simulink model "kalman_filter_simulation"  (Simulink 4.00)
settings: Solver=VariableStepDiscrete  StartTime=0.0  StopTime=100.0  RelTol=1e-3
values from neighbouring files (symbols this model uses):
  A = [1.1269   -0.4940    0.1129    [Kalman_Filter_Design_Example.m]
  Akf = kalmf.a    [Kalman_Filter_Design_Example.m]
  Ao = A - Ko*C    [Kalman_Filter_Design_Example.m]
  B = [-0.3832    [Kalman_Filter_Design_Example.m]
  Bkf = kalmf.b    [Kalman_Filter_Design_Example.m]
  Bo = [B Ko]    [Kalman_Filter_Design_Example.m]
  C = [1 0 0]    [Kalman_Filter_Design_Example.m]
  Ckf = kalmf.c    [Kalman_Filter_Design_Example.m]
  Co = C    [Kalman_Filter_Design_Example.m]
  D = zeros(1,2)    [Kalman_Filter_Design_Example.m]
  Dkf = kalmf.d    [Kalman_Filter_Design_Example.m]
  Do = zeros(1,2)    [Kalman_Filter_Design_Example.m]
  Tc = 1    [Kalman_Filter_Design_Example.m]

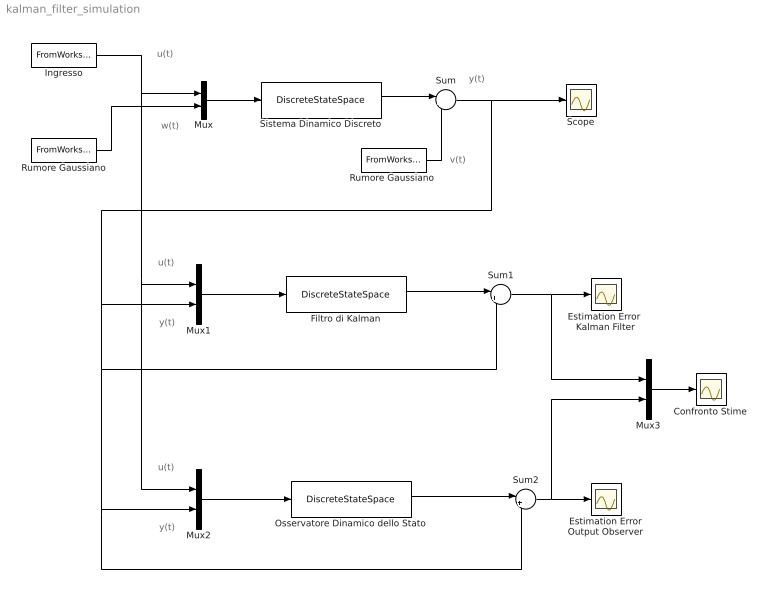
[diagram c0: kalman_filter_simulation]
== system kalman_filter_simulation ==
  note: u(t)
  note: w(t)
  note: y(t)
  note: v(t)
  note: u(t)
  note: y(t)
  note: u(t)
  note: y(t)
  Confronto Stime : Scope
  Estimation Error Output Observer : Scope
  Estimation Error  Kalman Filter : Scope
  Filtro di Kalman : DiscreteStateSpace  A=Akf  B=Bkf  C=Ckf  D=Dkf  X0=0  SampleTime=Tc  Realization=auto
  Ingresso : FromWorkspace  VariableName=[t u]  SampleTime=0  OutputAfterFinalValue=Extrapolation
  Mux{,1..3} (4 alike) : Mux  Inputs=2
  Osservatore Dinamico dello Stato : DiscreteStateSpace  A=Ao  B=Bo  C=Co  D=Do  X0=0  SampleTime=Tc  Realization=auto
  Rumore Gaussiano : FromWorkspace  VariableName=[t w]  SampleTime=Tc  OutputAfterFinalValue=Extrapolation
  "Rumore Gaussiano " : FromWorkspace  VariableName=[t v]  SampleTime=Tc  OutputAfterFinalValue=Extrapolation
  Scope : Scope
  Sistema Dinamico Discreto : DiscreteStateSpace  A=A  B=[B B]  C=C  D=D  X0=0  SampleTime=Tc  Realization=auto
  Sum : Sum  Inputs=|++  SaturateOnIntegerOverflow=on
  Sum1 : Sum  Inputs=|+-  SaturateOnIntegerOverflow=on
  Sum2 : Sum  Inputs=|+-  SaturateOnIntegerOverflow=on
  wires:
  Ingresso/1 -> Mux/1, Mux1/1, Mux2/1
  Rumore Gaussiano/1 -> Mux/2
  Mux/1 -> Sistema Dinamico Discreto/1
  Sistema Dinamico Discreto/1 -> Sum/1
  Sum/1 -> Scope/1, Mux1/2, Mux2/2, Sum2/2, Sum1/2
  "Rumore Gaussiano "/1 -> Sum/2
  Sum2/1 -> Estimation Error Output Observer/1, Mux3/2
  Sum1/1 -> Estimation Error  Kalman Filter/1, Mux3/1
  Mux3/1 -> Confronto Stime/1
  Mux2/1 -> Osservatore Dinamico dello Stato/1
  Osservatore Dinamico dello Stato/1 -> Sum2/1
  Mux1/1 -> Filtro di Kalman/1
  Filtro di Kalman/1 -> Sum1/1
